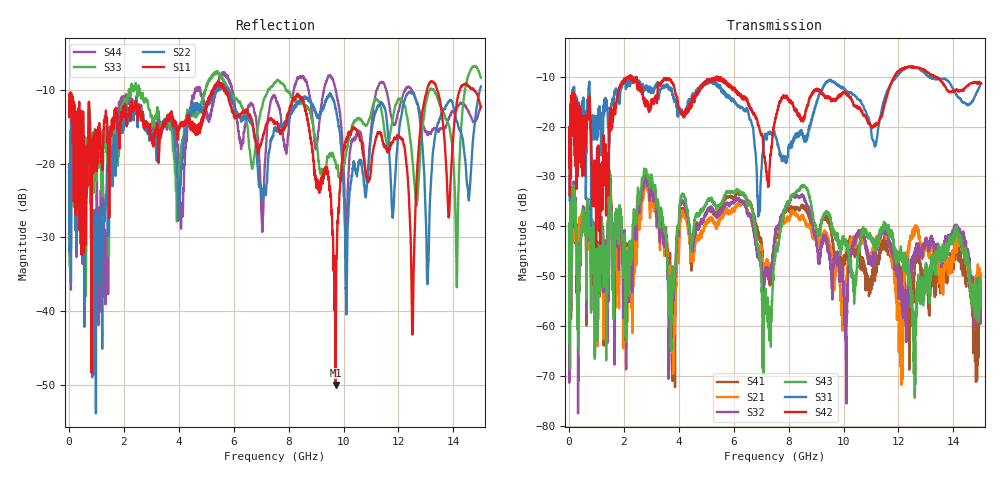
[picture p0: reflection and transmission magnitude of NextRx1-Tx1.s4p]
! FILE: N:\QM 2007\Prüfprotokolle\Highspeed\Konfektionierte Ltg\L45593-D106\D30\8216\0002\Next  Platine 2\NextRx1-Tx1.s4p
# MHz S DB R 50.00
! FREQ  S11  S12  S13  S14
!  S21  S22  S23  S24
!  S31  S32  S33  S34
!  S41  S42  S43  S44
!  DB  ANG  DB  ANG  DB  ANG  DB  ANG
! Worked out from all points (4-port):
!   2999 points, 10 MHz to 15 GHz, reference 50 ohm
!   strongest paths, dB at 10 MHz, 3.755 GHz, 7.505 GHz, 11.26 GHz, 15 GHz:
!     S42: -24.3, -11.1, -18.9, -19.3, -11.4
!     S31: -26.1, -12.5, -21.6, -20.6, -11.4
!     S43: -48.3, -55.1, -45.7, -43.2, -52.3
!     S32: -44.9, -50.5, -41.9, -43.5, -53.8
!     S21: -54.5, -55.0, -42.0, -42.0, -51.4
!     S41: -51.6, -57.4, -44.1, -45.9, -53.8
!   lowest |S11| = -50.1 dB at 9.715 GHz (marker M1), VSWR 1.01, Z = 50.1 - j0.308 ohm
!   |S11| at or under -10 dB: start of sweep to 5.222 GHz; 5.704 GHz to 13.03 GHz (7.33 GHz wide, 78.2 % of centre); 13.41 GHz to 14.23 GHz (816.2 MHz wide, 5.91 % of centre)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
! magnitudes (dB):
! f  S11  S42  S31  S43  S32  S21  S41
! 10 MHz  -11.5  -24.3  -26.1  -48.3  -44.9  -54.5  -51.6
! 3.805 GHz  -13.9  -11.7  -14.5  -50.8  -51.7  -69.2  -59.5
! 6.15 GHz  -13.5  -13.5  -15.9  -32.9  -34.4  -35.5  -33.5
! 7.3 GHz  -14.0  -28.8  -21.3  -62.8  -50.2  -48.0  -51.7
! 8.375 GHz  -10.8  -17.9  -22.0  -32.8  -34.4  -38.2  -36.5
! 9.715 GHz  -50.1  -14.5  -11.3  -42.7  -46.3  -49.6  -48.6
! 15 GHz  -12.3  -11.4  -11.4  -52.3  -53.8  -51.4  -53.8
